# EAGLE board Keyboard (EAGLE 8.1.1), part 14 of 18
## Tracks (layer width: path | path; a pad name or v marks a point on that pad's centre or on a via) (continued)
S$14353
  Bottom 0: 155.42,84.92 155.38,84.86
S$14354
  Bottom 0: 155.38,84.86 155.35,84.8
S$14355
  Bottom 0: 155.35,84.8 155.34,84.73
S$14356
  Bottom 0: 155.34,84.73 155.33,84.66
S$14357
  Bottom 0: 155.33,84.66 155.33,76.26
S$14358
  Bottom 0: 155.33,76.26 155.24,76.17
S$14359
  Bottom 0: 155.24,76.17 155.06,75.89
S$14360
  Bottom 0: 155.06,75.89 154.98,75.58
S$14361
  Bottom 0: 154.98,75.58 154.98,75.26
S$14362
  Bottom 0: 154.98,75.26 155.06,74.94
S$14363
  Bottom 0: 155.06,74.94 155.24,74.67
S$14364
  Bottom 0: 155.24,74.67 155.47,74.44
S$14365
  Bottom 0: 155.47,74.44 155.76,74.3
S$14366
  Bottom 0: 155.76,74.3 156.08,74.23
S$14367
  Bottom 0: 156.08,74.23 156.41,74.25
S$14368
  Bottom 0: 156.41,74.25 156.71,74.36
S$14369
  Bottom 0: 156.71,74.36 156.97,74.55
S$14370
  Bottom 0: 156.97,74.55 157.18,74.8
S$14371
  Bottom 0: 157.18,74.8 157.31,75.1
S$14372
  Bottom 0: 157.31,75.1 157.36,75.42
S$14373
  Bottom 0: 157.36,75.42 157.31,75.74
S$14374
  Bottom 0: 157.31,75.74 157.18,76.04
S$14375
  Bottom 0: 157.18,76.04 156.97,76.29
S$14376
  Bottom 0: 156.97,76.29 156.71,76.48
S$14377
  Bottom 0: 156.71,76.48 156.41,76.59
S$14378
  Bottom 0: 156.41,76.59 156.22,76.6
S$14379
  Bottom 0: 156.22,76.6 156.22,77.98
S$14380
  Bottom 0: 156.22,77.98 156.29,77.85
S$14381
  Bottom 0: 156.29,77.85 156.53,77.6
S$14382
  Bottom 0: 156.53,77.6 156.82,77.41
S$14383
  Bottom 0: 156.82,77.41 157.15,77.31
S$14384
  Bottom 0: 157.15,77.31 157.5,77.28
S$14385
  Bottom 0: 157.5,77.28 157.85,77.35
S$14386
  Bottom 0: 157.85,77.35 158.16,77.5
S$14387
  Bottom 0: 158.16,77.5 158.43,77.72
S$14388
  Bottom 0: 158.43,77.72 158.64,78.01
S$14389
  Bottom 0: 158.64,78.01 158.77,78.33
S$14390
  Bottom 0: 158.77,78.33 158.81,78.68
S$14391
  Bottom 0: 158.81,78.68 158.77,79.02
S$14392
  Bottom 0: 158.77,79.02 158.64,79.35
S$14393
  Bottom 0: 158.64,79.35 158.43,79.63
S$14394
  Bottom 0: 158.43,79.63 158.16,79.86
S$14395
  Bottom 0: 158.16,79.86 157.85,80.01
S$14396
  Bottom 0: 157.85,80.01 157.5,80.07
S$14397
  Bottom 0: 157.5,80.07 157.15,80.05
S$14398
  Bottom 0: 157.15,80.05 156.82,79.94
S$14399
  Bottom 0: 156.82,79.94 156.53,79.75
S$14400
  Bottom 0: 156.53,79.75 156.29,79.5
S$14401
  Bottom 0: 156.29,79.5 156.22,79.37
S$14402
  Bottom 0: 156.22,79.37 156.22,84.48
S$14403
  Bottom 0: 156.22,84.48 159,87.25
S$14404
  Bottom 0: 159,87.25 159.03,87.31
S$14405
  Bottom 0: 159.03,87.31 159.07,87.35
S$14406
  Bottom 0: 159.07,87.35 159.08,87.39
S$14407
  Bottom 0: 159.08,87.39 159.11,87.45
S$14408
  Bottom 0: 159.11,87.45 159.11,87.51
S$14409
  Bottom 0: 159.11,87.51 159.13,87.57
S$14410
  Bottom 0: 159.13,87.57 159.13,87.69
S$14411
  Bottom 0: 159.13,87.69 159.58,87.69
S$14412
  Bottom 0: 159.58,87.69 159.65,87.7
S$14413
  Bottom 0: 159.65,87.7 159.72,87.74
S$14414
  Bottom 0: 159.72,87.74 159.78,87.8
S$14415
  Bottom 0: 159.78,87.8 159.82,87.87
S$14416
  Bottom 0: 159.82,87.87 159.83,87.95
S$14417
  Bottom 0: 159.83,87.95 159.83,89.65
S$14418
  Bottom 0: 159.83,89.65 160.44,89.65
S$14419
  Bottom 0: 160.44,89.65 160.27,89.46
S$14420
  Bottom 0: 160.27,89.46 160.13,89.16
S$14421
  Bottom 0: 160.13,89.16 160.08,88.84
S$14422
  Bottom 0: 160.08,88.84 160.13,88.52
S$14423
  Bottom 0: 160.13,88.52 160.27,88.22
S$14424
  Bottom 0: 160.27,88.22 160.48,87.97
S$14425
  Bottom 0: 160.48,87.97 160.75,87.8
S$14426
  Bottom 0: 160.75,87.8 161.06,87.7
S$14427
  Bottom 0: 161.06,87.7 161.39,87.7
S$14428
  Bottom 0: 161.39,87.7 161.52,87.74
S$14429
  Bottom 0: 161.52,87.74 161.91,87.35
S$14430
  Bottom 0: 161.91,87.35 161.91,84.92
S$14431
  Bottom 0: 161.91,84.92 161.86,85.03
S$14432
  Bottom 0: 161.86,85.03 161.57,85.37
S$14433
  Bottom 0: 161.57,85.37 161.23,85.66
S$14434
  Bottom 0: 161.23,85.66 160.83,85.87
S$14435
  Bottom 0: 160.83,85.87 160.4,86
S$14436
  Bottom 0: 160.4,86 159.96,86.04
S$14437
  Bottom 0: 159.96,86.04 159.51,86
S$14438
  Bottom 0: 159.51,86 159.08,85.87
S$14439
  Bottom 0: 159.08,85.87 158.69,85.66
S$14440
  Bottom 0: 158.69,85.66 158.34,85.37
S$14441
  Bottom 0: 158.34,85.37 158.06,85.03
S$14442
  Bottom 0: 158.06,85.03 157.84,84.63
S$14443
  Bottom 0: 157.84,84.63 157.71,84.2
S$14444
  Bottom 0: 157.71,84.2 157.67,83.76
S$14445
  Bottom 0: 157.67,83.76 157.71,83.31
S$14446
  Bottom 0: 157.71,83.31 157.84,82.88
S$14447
  Bottom 0: 157.84,82.88 158.06,82.49
S$14448
  Bottom 0: 158.06,82.49 158.34,82.14
S$14449
  Bottom 0: 158.34,82.14 158.69,81.86
S$14450
  Bottom 0: 158.69,81.86 159.08,81.64
S$14451
  Bottom 0: 159.08,81.64 159.51,81.52
S$14452
  Bottom 0: 159.51,81.52 159.96,81.47
S$14453
  Bottom 0: 159.96,81.47 160.4,81.52
S$14454
  Bottom 0: 160.4,81.52 160.83,81.64
S$14455
  Bottom 0: 160.83,81.64 161.23,81.86
S$14456
  Bottom 0: 161.23,81.86 161.43,82.02
S$14457
  Bottom 0: 161.43,82.02 161.43,73.36
S$14458
  Bottom 0: 161.43,73.36 161.43,73.27
S$14459
  Bottom 0: 161.43,73.27 161.45,73.19
S$14460
  Bottom 0: 161.45,73.19 161.49,73.1
S$14461
  Bottom 0: 161.49,73.1 161.53,73.03
S$14462
  Bottom 0: 161.53,73.03 161.59,72.96
S$14463
  Bottom 0: 161.59,72.96 166.56,68
S$14464
  Bottom 0: 166.56,68 166.62,67.94
S$14465
  Bottom 0: 166.62,67.94 166.7,67.89
S$14466
  Bottom 0: 166.7,67.89 166.78,67.86
S$14467
  Bottom 0: 166.78,67.86 166.87,67.83
S$14468
  Bottom 0: 166.87,67.83 166.96,67.83
S$14469
  Bottom 0: 166.96,67.83 169.37,67.83
S$14470
  Bottom 0: 169.37,67.83 169.46,67.83
S$14471
  Bottom 0: 169.46,67.83 169.54,67.86
S$14472
  Bottom 0: 169.54,67.86 169.62,67.89
S$14473
  Bottom 0: 169.62,67.89 169.7,67.94
S$14474
  Bottom 0: 169.7,67.94 169.76,68
S$14475
  Bottom 0: 169.76,68 170.46,68.69
S$14476
  Bottom 0: 170.46,68.69 170.59,68.65
S$14477
  Bottom 0: 170.59,68.65 170.91,68.65
S$14478
  Bottom 0: 170.91,68.65 171.22,68.75
S$14479
  Bottom 0: 171.22,68.75 171.5,68.92
S$14480
  Bottom 0: 171.5,68.92 171.71,69.16
S$14481
  Bottom 0: 171.71,69.16 171.85,69.47
S$14482
  Bottom 0: 171.85,69.47 171.89,69.79
S$14483
  Bottom 0: 171.89,69.79 171.85,70.11
S$14484
  Bottom 0: 171.85,70.11 171.71,70.41
S$14485
  Bottom 0: 171.71,70.41 171.5,70.65
S$14486
  Bottom 0: 171.5,70.65 171.22,70.83
S$14487
  Bottom 0: 171.22,70.83 170.91,70.92
S$14488
  Bottom 0: 170.91,70.92 170.59,70.92
S$14489
  Bottom 0: 170.59,70.92 170.28,70.83
S$14490
  Bottom 0: 170.28,70.83 170,70.65
S$14491
  Bottom 0: 170,70.65 169.79,70.41
S$14492
  Bottom 0: 169.79,70.41 169.65,70.11
S$14493
  Bottom 0: 169.65,70.11 169.61,69.79
S$14494
  Bottom 0: 169.61,69.79 169.65,69.48
S$14495
  Bottom 0: 169.65,69.48 169.35,69.19
S$14496
  Bottom 0: 169.35,69.19 169.35,70.67
S$14497
  Bottom 0: 169.35,70.67 169.34,70.75
S$14498
  Bottom 0: 169.34,70.75 169.3,70.82
S$14499
  Bottom 0: 169.3,70.82 169.25,70.88
S$14500
  Bottom 0: 169.25,70.88 169.18,70.92
S$14501
  Bottom 0: 169.18,70.92 169.1,70.93
S$14502
  Bottom 0: 169.1,70.93 168.65,70.93
S$14503
  Bottom 0: 168.65,70.93 168.65,71.06
S$14504
  Bottom 0: 168.65,71.06 168.59,71.28
S$14505
  Bottom 0: 168.59,71.28 168.43,71.44
S$14506
  Bottom 0: 168.43,71.44 168.21,71.5
S$14507
  Bottom 0: 168.21,71.5 167.86,71.5
S$14508
  Bottom 0: 167.86,71.5 166.77,72.58
S$14509
  Bottom 0: 166.77,72.58 166.84,72.72
S$14510
  Bottom 0: 166.84,72.72 166.88,73.04
S$14511
  Bottom 0: 166.88,73.04 166.84,73.36
S$14512
  Bottom 0: 166.84,73.36 166.71,73.66
S$14513
  Bottom 0: 166.71,73.66 166.5,73.92
S$14514
  Bottom 0: 166.5,73.92 166.24,74.11
S$14515
  Bottom 0: 166.24,74.11 165.93,74.21
S$14516
  Bottom 0: 165.93,74.21 165.6,74.23
S$14517
  Bottom 0: 165.6,74.23 165.28,74.17
S$14518
  Bottom 0: 165.28,74.17 165,74.02
S$14519
  Bottom 0: 165,74.02 164.76,73.8
S$14520
  Bottom 0: 164.76,73.8 164.59,73.52
S$14521
  Bottom 0: 164.59,73.52 164.5,73.2
S$14522
  Bottom 0: 164.5,73.2 164.5,72.88
S$14523
  Bottom 0: 164.5,72.88 164.59,72.56
S$14524
  Bottom 0: 164.59,72.56 164.76,72.29
S$14525
  Bottom 0: 164.76,72.29 165,72.07
S$14526
  Bottom 0: 165,72.07 165.28,71.92
S$14527
  Bottom 0: 165.28,71.92 165.6,71.85
S$14528
  Bottom 0: 165.6,71.85 165.93,71.87
S$14529
  Bottom 0: 165.93,71.87 166.15,71.95
S$14530
  Bottom 0: 166.15,71.95 167.21,70.9
S$14531
  Bottom 0: 167.21,70.9 167.18,70.88
S$14532
  Bottom 0: 167.18,70.88 167.12,70.82
S$14533
  Bottom 0: 167.12,70.82 167.08,70.75
S$14534
  Bottom 0: 167.08,70.75 167.07,70.67
S$14535
  Bottom 0: 167.07,70.67 167.07,69.09
S$14536
  Bottom 0: 167.07,69.09 162.56,73.6
S$14537
  Bottom 0: 162.56,73.6 162.56,80.53
S$14538
  Bottom 0: 162.56,80.53 162.64,80.39
S$14539
  Bottom 0: 162.64,80.39 162.88,80.14
S$14540
  Bottom 0: 162.88,80.14 163.17,79.95
S$14541
  Bottom 0: 163.17,79.95 163.5,79.84
S$14542
  Bottom 0: 163.5,79.84 163.85,79.83
S$14543
  Bottom 0: 163.85,79.83 164.2,79.89
S$14544
  Bottom 0: 164.2,79.89 164.38,79.97
S$14545
  Bottom 0: 164.38,79.97 167.75,76.6
S$14546
  Bottom 0: 167.75,76.6 167.81,76.56
S$14547
  Bottom 0: 167.81,76.56 167.87,76.52
S$14548
  Bottom 0: 167.87,76.52 167.93,76.5
S$14549
  Bottom 0: 167.93,76.5 167.99,76.48
S$14550
  Bottom 0: 167.99,76.48 168.06,76.48
S$14551
  Bottom 0: 168.06,76.48 171.65,76.48
S$14552
  Bottom 0: 171.65,76.48 174.33,73.79
S$14553
  Bottom 0: 174.33,73.79 174.39,73.75
S$14554
  Bottom 0: 174.39,73.75 174.45,73.71
S$14555
  Bottom 0: 174.45,73.71 174.51,73.68
S$14556
  Bottom 0: 174.51,73.68 174.58,73.67
S$14557
  Bottom 0: 174.58,73.67 174.65,73.66
S$14558
  Bottom 0: 174.65,73.66 178.43,73.66
S$14559
  Bottom 0: 178.43,73.66 178.5,73.67
S$14560
  Bottom 0: 178.5,73.67 178.57,73.68
S$14561
  Bottom 0: 178.57,73.68 178.63,73.71
S$14562
  Bottom 0: 178.63,73.71 178.69,73.75
S$14563
  Bottom 0: 178.69,73.75 178.75,73.79
S$14564
  Bottom 0: 178.75,73.79 181.28,76.32
S$14565
  Bottom 0: 181.28,76.32 182.07,76.32
S$14566
  Bottom 0: 182.07,76.32 181.91,76.17
S$14567
  Bottom 0: 181.91,76.17 181.74,75.89
S$14568
  Bottom 0: 181.74,75.89 181.65,75.58
S$14569
  Bottom 0: 181.65,75.58 181.65,75.25
S$14570
  Bottom 0: 181.65,75.25 181.7,75.08
S$14571
  Bottom 0: 181.7,75.08 180.23,73.61
S$14572
  Bottom 0: 180.23,73.61 174.35,73.61
S$14573
  Bottom 0: 174.35,73.61 174.33,73.66
S$14574
  Bottom 0: 174.33,73.66 174.12,73.92
S$14575
  Bottom 0: 174.12,73.92 173.85,74.11
S$14576
  Bottom 0: 173.85,74.11 173.55,74.21
S$14577
  Bottom 0: 173.55,74.21 173.22,74.23
S$14578
  Bottom 0: 173.22,74.23 172.98,74.18
S$14579
  Bottom 0: 172.98,74.18 171.34,75.82
S$14580
  Bottom 0: 171.34,75.82 171.27,75.88
S$14581
  Bottom 0: 171.27,75.88 171.19,75.93
S$14582
  Bottom 0: 171.19,75.93 171.11,75.96
S$14583
  Bottom 0: 171.11,75.96 171.03,75.98
S$14584
  Bottom 0: 171.03,75.98 170.93,75.99
S$14585
  Bottom 0: 170.93,75.99 164.82,75.99
S$14586
  Bottom 0: 164.82,75.99 164.8,76.04
S$14587
  Bottom 0: 164.8,76.04 164.59,76.29
S$14588
  Bottom 0: 164.59,76.29 164.33,76.48
S$14589
  Bottom 0: 164.33,76.48 164.03,76.59
S$14590
  Bottom 0: 164.03,76.59 163.7,76.61
S$14591
  Bottom 0: 163.7,76.61 163.38,76.54
S$14592
  Bottom 0: 163.38,76.54 163.09,76.4
S$14593
  Bottom 0: 163.09,76.4 162.85,76.17
S$14594
  Bottom 0: 162.85,76.17 162.68,75.89
S$14595
  Bottom 0: 162.68,75.89 162.6,75.58
S$14596
  Bottom 0: 162.6,75.58 162.6,75.26
S$14597
  Bottom 0: 162.6,75.26 162.68,74.94
S$14598
  Bottom 0: 162.68,74.94 162.85,74.67
S$14599
  Bottom 0: 162.85,74.67 163.09,74.44
S$14600
  Bottom 0: 163.09,74.44 163.38,74.3
S$14601
  Bottom 0: 163.38,74.3 163.7,74.23
S$14602
  Bottom 0: 163.7,74.23 164.03,74.25
S$14603
  Bottom 0: 164.03,74.25 164.33,74.36
S$14604
  Bottom 0: 164.33,74.36 164.59,74.55
S$14605
  Bottom 0: 164.59,74.55 164.8,74.8
S$14606
  Bottom 0: 164.8,74.8 164.82,74.85
S$14607
  Bottom 0: 164.82,74.85 170.7,74.85
S$14608
  Bottom 0: 170.7,74.85 172.17,73.38
S$14609
  Bottom 0: 172.17,73.38 172.12,73.2
S$14610
  Bottom 0: 172.12,73.2 172.12,72.88
S$14611
  Bottom 0: 172.12,72.88 172.21,72.56
S$14612
  Bottom 0: 172.21,72.56 172.38,72.29
S$14613
  Bottom 0: 172.38,72.29 172.61,72.07
S$14614
  Bottom 0: 172.61,72.07 172.91,71.92
S$14615
  Bottom 0: 172.91,71.92 173.22,71.85
S$14616
  Bottom 0: 173.22,71.85 173.55,71.87
S$14617
  Bottom 0: 173.55,71.87 173.85,71.98
S$14618
  Bottom 0: 173.85,71.98 174.12,72.17
S$14619
  Bottom 0: 174.12,72.17 174.33,72.42
S$14620
  Bottom 0: 174.33,72.42 174.35,72.47
S$14621
  Bottom 0: 174.35,72.47 180.46,72.47
S$14622
  Bottom 0: 180.46,72.47 180.55,72.48
S$14623
  Bottom 0: 180.55,72.48 180.64,72.5
S$14624
  Bottom 0: 180.64,72.5 180.72,72.53
S$14625
  Bottom 0: 180.72,72.53 180.8,72.58
S$14626
  Bottom 0: 180.8,72.58 180.87,72.64
S$14627
  Bottom 0: 180.87,72.64 182.5,74.28
S$14628
  Bottom 0: 182.5,74.28 182.76,74.23
S$14629
  Bottom 0: 182.76,74.23 183.08,74.24
S$14630
  Bottom 0: 183.08,74.24 183.38,74.35
S$14631
  Bottom 0: 183.38,74.35 183.65,74.54
S$14632
  Bottom 0: 183.65,74.54 183.85,74.8
S$14633
  Bottom 0: 183.85,74.8 183.88,74.84
S$14634
  Bottom 0: 183.88,74.84 189.76,74.84
S$14635
  Bottom 0: 189.76,74.84 191.22,73.38
S$14636
  Bottom 0: 191.22,73.38 191.18,73.2
S$14637
  Bottom 0: 191.18,73.2 191.18,72.88
S$14638
  Bottom 0: 191.18,72.88 191.26,72.56
S$14639
  Bottom 0: 191.26,72.56 191.44,72.29
S$14640
  Bottom 0: 191.44,72.29 191.67,72.07
S$14641
  Bottom 0: 191.67,72.07 191.96,71.92
S$14642
  Bottom 0: 191.96,71.92 192.28,71.85
S$14643
  Bottom 0: 192.28,71.85 192.61,71.87
S$14644
  Bottom 0: 192.61,71.87 192.91,71.98
S$14645
  Bottom 0: 192.91,71.98 193.18,72.17
S$14646
  Bottom 0: 193.18,72.17 193.38,72.42
S$14647
  Bottom 0: 193.38,72.42 193.51,72.72
S$14648
  Bottom 0: 193.51,72.72 193.56,73.04
S$14649
  Bottom 0: 193.56,73.04 193.52,73.29
S$14650
  Bottom 0: 193.52,73.29 194.4,72.41
S$14651
  Bottom 0: 194.4,72.41 194.46,72.37
S$14652
  Bottom 0: 194.46,72.37 194.52,72.33
S$14653
  Bottom 0: 194.52,72.33 194.58,72.3
S$14654
  Bottom 0: 194.58,72.3 194.64,72.29
S$14655
  Bottom 0: 194.64,72.29 194.71,72.28
S$14656
  Bottom 0: 194.71,72.28 200.03,72.28
S$14657
  Bottom 0: 200.03,72.28 204.76,67.55
S$14658
  Bottom 0: 204.76,67.55 204.81,67.51
S$14659
  Bottom 0: 204.81,67.51 204.87,67.47
S$14660
  Bottom 0: 204.87,67.47 204.94,67.44
S$14661
  Bottom 0: 204.94,67.44 205,67.43
S$14662
  Bottom 0: 205,67.43 205.07,67.42
S$14663
  Bottom 0: 205.07,67.42 207.63,67.42
S$14664
  Bottom 0: 207.63,67.42 208.13,66.92
S$14665
  Bottom 0: 208.13,66.92 208.03,66.94
S$14666
  Bottom 0: 208.03,66.94 207.58,66.99
S$14667
  Bottom 0: 207.58,66.99 207.13,66.94
S$14668
  Bottom 0: 207.13,66.94 206.71,66.82
S$14669
  Bottom 0: 206.71,66.82 206.31,66.61
S$14670
  Bottom 0: 206.31,66.61 205.97,66.32
S$14671
  Bottom 0: 205.97,66.32 205.68,65.98
S$14672
  Bottom 0: 205.68,65.98 205.47,65.58
S$14673
  Bottom 0: 205.47,65.58 205.34,65.15
S$14674
  Bottom 0: 205.34,65.15 205.3,64.71
S$14675
  Bottom 0: 205.3,64.71 205.34,64.26
S$14676
  Bottom 0: 205.34,64.26 205.47,63.83
S$14677
  Bottom 0: 205.47,63.83 205.68,63.44
S$14678
  Bottom 0: 205.68,63.44 205.97,63.09
S$14679
  Bottom 0: 205.97,63.09 206.31,62.81
S$14680
  Bottom 0: 206.31,62.81 206.71,62.59
S$14681
  Bottom 0: 206.71,62.59 207.13,62.47
S$14682
  Bottom 0: 207.13,62.47 207.58,62.42
S$14683
  Bottom 0: 207.58,62.42 208.03,62.47
S$14684
  Bottom 0: 208.03,62.47 208.46,62.59
S$14685
  Bottom 0: 208.46,62.59 208.85,62.81
S$14686
  Bottom 0: 208.85,62.81 209.19,63.09
S$14687
  Bottom 0: 209.19,63.09 209.48,63.44
S$14688
  Bottom 0: 209.48,63.44 209.69,63.83
S$14689
  Bottom 0: 209.69,63.83 209.82,64.26
S$14690
  Bottom 0: 209.82,64.26 209.87,64.71
S$14691
  Bottom 0: 209.87,64.71 209.82,65.15
S$14692
  Bottom 0: 209.82,65.15 209.79,65.26
S$14693
  Bottom 0: 209.79,65.26 211.5,63.55
S$14694
  Bottom 0: 211.5,63.55 211.47,63.56
S$14695
  Bottom 0: 211.47,63.56 211.13,63.54
S$14696
  Bottom 0: 211.13,63.54 210.8,63.43
S$14697
  Bottom 0: 210.8,63.43 210.5,63.24
S$14698
  Bottom 0: 210.5,63.24 210.26,62.99
S$14699
  Bottom 0: 210.26,62.99 210.09,62.68
S$14700
  Bottom 0: 210.09,62.68 210,62.34
S$14701
  Bottom 0: 210,62.34 210,61.99
S$14702
  Bottom 0: 210,61.99 210.09,61.65
S$14703
  Bottom 0: 210.09,61.65 210.26,61.34
S$14704
  Bottom 0: 210.26,61.34 210.5,61.09
S$14705
  Bottom 0: 210.5,61.09 210.8,60.9
S$14706
  Bottom 0: 210.8,60.9 211.13,60.8
S$14707
  Bottom 0: 211.13,60.8 211.47,60.77
S$14708
  Bottom 0: 211.47,60.77 211.82,60.84
S$14709
  Bottom 0: 211.82,60.84 212.14,60.99
S$14710
  Bottom 0: 212.14,60.99 212.41,61.21
S$14711
  Bottom 0: 212.41,61.21 212.62,61.5
S$14712
  Bottom 0: 212.62,61.5 212.74,61.82
S$14713
  Bottom 0: 212.74,61.82 212.79,62.17
S$14714
  Bottom 0: 212.79,62.17 212.77,62.28
S$14715
  Bottom 0: 212.77,62.28 223.37,51.68
S$14716
  Bottom 0: 223.37,51.68 223.43,51.64
S$14717
  Bottom 0: 223.43,51.64 223.48,51.6
S$14718
  Bottom 0: 223.48,51.6 223.54,51.57
S$14719
  Bottom 0: 223.54,51.57 223.61,51.56
S$14720
  Bottom 0: 223.61,51.56 223.69,51.55
S$14721
  Bottom 0: 223.69,51.55 228.98,51.55
S$14722
  Bottom 0: 228.98,51.55 228.98,49.84
S$14723
  Bottom 0: 228.98,49.84 222.88,49.84
S$14724
  Bottom 0: 222.88,49.84 222.86,50
S$14725
  Bottom 0: 222.86,50 222.72,50.27
S$14726
  Bottom 0: 222.72,50.27 222.52,50.49
S$14727
  Bottom 0: 222.52,50.49 222.26,50.65
S$14728
  Bottom 0: 222.26,50.65 221.96,50.71
S$14729
  Bottom 0: 221.96,50.71 221.66,50.69
S$14730
  Bottom 0: 221.66,50.69 221.38,50.58
S$14731
  Bottom 0: 221.38,50.58 221.14,50.39
S$14732
  Bottom 0: 221.14,50.39 220.97,50.14
S$14733
  Bottom 0: 220.97,50.14 220.88,49.85
S$14734
  Bottom 0: 220.88,49.85 220.88,49.55
S$14735
  Bottom 0: 220.88,49.55 220.97,49.26
S$14736
  Bottom 0: 220.97,49.26 221.14,49.01
S$14737
  Bottom 0: 221.14,49.01 221.38,48.82
S$14738
  Bottom 0: 221.38,48.82 221.66,48.71
S$14739
  Bottom 0: 221.66,48.71 221.96,48.69
S$14740
  Bottom 0: 221.96,48.69 222.26,48.76
S$14741
  Bottom 0: 222.26,48.76 222.52,48.91
S$14742
  Bottom 0: 222.52,48.91 222.56,48.95
S$14743
  Bottom 0: 222.56,48.95 240.27,48.95
S$14744
  Bottom 0: 240.27,48.95 240.43,48.82
S$14745
  Bottom 0: 240.43,48.82 240.71,48.71
S$14746
  Bottom 0: 240.71,48.71 241.02,48.69
S$14747
  Bottom 0: 241.02,48.69 241.31,48.76
S$14748
  Bottom 0: 241.31,48.76 241.57,48.91
S$14749
  Bottom 0: 241.57,48.91 241.78,49.13
S$14750
  Bottom 0: 241.78,49.13 241.91,49.4
S$14751
  Bottom 0: 241.91,49.4 241.96,49.7
S$14752
  Bottom 0: 241.96,49.7 241.91,50
S$14753
  Bottom 0: 241.91,50 241.78,50.27
S$14754
  Bottom 0: 241.78,50.27 241.57,50.49
S$14755
  Bottom 0: 241.57,50.49 241.31,50.65
S$14756
  Bottom 0: 241.31,50.65 241.02,50.71
S$14757
  Bottom 0: 241.02,50.71 240.71,50.69
S$14758
  Bottom 0: 240.71,50.69 240.43,50.58
S$14759
  Bottom 0: 240.43,50.58 240.19,50.39
S$14760
  Bottom 0: 240.19,50.39 240.03,50.14
S$14761
  Bottom 0: 240.03,50.14 239.94,49.85
S$14762
  Bottom 0: 239.94,49.85 239.94,49.84
S$14763
  Bottom 0: 239.94,49.84 233.35,49.84
S$14764
  Bottom 0: 233.35,49.84 233.41,49.87
S$14765
  Bottom 0: 233.41,49.87 233.62,50.11
S$14766
  Bottom 0: 233.62,50.11 233.76,50.42
S$14767
  Bottom 0: 233.76,50.42 233.8,50.74
S$14768
  Bottom 0: 233.8,50.74 233.76,51.06
S$14769
  Bottom 0: 233.76,51.06 233.62,51.36
S$14770
  Bottom 0: 233.62,51.36 233.45,51.55
S$14771
  Bottom 0: 233.45,51.55 240.78,51.55
S$14772
  Bottom 0: 240.78,51.55 242.49,49.84
S$14773
  Bottom 0: 242.49,49.84 242.49,49.67
S$14774
  Bottom 0: 242.49,49.67 242.53,49.54
S$14775
  Bottom 0: 242.53,49.54 242.43,49.53
S$14776
  Bottom 0: 242.43,49.53 242.21,49.41
S$14777
  Bottom 0: 242.21,49.41 242.03,49.23
S$14778
  Bottom 0: 242.03,49.23 241.94,48.99
S$14779
  Bottom 0: 241.94,48.99 241.94,48.74
S$14780
  Bottom 0: 241.94,48.74 242.03,48.51
S$14781
  Bottom 0: 242.03,48.51 242.08,48.46
S$14782
  Bottom 0: 242.08,48.46 236.58,42.96
S$14783
  Bottom 0: 179.09,67.74 179.39,67.81
S$14784
  Bottom 0: 179.39,67.81 179.66,67.95
S$14785
  Bottom 0: 179.66,67.95 179.86,68.18
S$14786
  Bottom 0: 179.86,68.18 179.99,68.45
S$14787
  Bottom 0: 179.99,68.45 180.04,68.75
S$14788
  Bottom 0: 180.04,68.75 179.99,69.05
S$14789
  Bottom 0: 179.99,69.05 179.86,69.32
S$14790
  Bottom 0: 179.86,69.32 179.66,69.54
S$14791
  Bottom 0: 179.66,69.54 179.39,69.69
S$14792
  Bottom 0: 179.39,69.69 179.09,69.76
S$14793
  Bottom 0: 179.09,69.76 178.79,69.74
S$14794
  Bottom 0: 178.79,69.74 178.51,69.63
S$14795
  Bottom 0: 178.51,69.63 178.27,69.44
S$14796
  Bottom 0: 178.27,69.44 178.11,69.19
S$14797
  Bottom 0: 178.11,69.19 178.01,68.9
S$14798
  Bottom 0: 178.01,68.9 178.01,68.59
S$14799
  Bottom 0: 178.01,68.59 178.11,68.31
S$14800
  Bottom 0: 178.11,68.31 178.27,68.06
S$14801
  Bottom 0: 178.27,68.06 178.51,67.87
S$14802
  Bottom 0: 178.51,67.87 178.79,67.76
S$14803
  Bottom 0: 178.79,67.76 179.09,67.74
S$14804
  Bottom 0: 160.05,67.74 160.34,67.81
S$14805
  Bottom 0: 160.34,67.81 160.6,67.95
S$14806
  Bottom 0: 160.6,67.95 160.81,68.18
S$14807
  Bottom 0: 160.81,68.18 160.94,68.45
S$14808
  Bottom 0: 160.94,68.45 160.99,68.75
S$14809
  Bottom 0: 160.99,68.75 160.94,69.05
S$14810
  Bottom 0: 160.94,69.05 160.81,69.32
S$14811
  Bottom 0: 160.81,69.32 160.6,69.54
S$14812
  Bottom 0: 160.6,69.54 160.34,69.69
S$14813
  Bottom 0: 160.34,69.69 160.05,69.76
S$14814
  Bottom 0: 160.05,69.76 159.74,69.74
S$14815
  Bottom 0: 159.74,69.74 159.46,69.63
S$14816
  Bottom 0: 159.46,69.63 159.22,69.44
S$14817
  Bottom 0: 159.22,69.44 159.06,69.19
S$14818
  Bottom 0: 159.06,69.19 158.97,68.9
S$14819
  Bottom 0: 158.97,68.9 158.97,68.59
S$14820
  Bottom 0: 158.97,68.59 159.06,68.31
S$14821
  Bottom 0: 159.06,68.31 159.22,68.06
S$14822
  Bottom 0: 159.22,68.06 159.46,67.87
S$14823
  Bottom 0: 159.46,67.87 159.74,67.76
S$14824
  Bottom 0: 159.74,67.76 160.05,67.74
S$14825
  Bottom 0: 186.37,68.64 188.15,68.64
S$14826
  Bottom 0: 188.15,68.64 188.23,68.65
S$14827
  Bottom 0: 188.23,68.65 188.3,68.69
S$14828
  Bottom 0: 188.3,68.69 188.35,68.75
S$14829
  Bottom 0: 188.35,68.75 188.39,68.82
S$14830
  Bottom 0: 188.39,68.82 188.41,68.9
S$14831
  Bottom 0: 188.41,68.9 188.41,70.67
S$14832
  Bottom 0: 188.41,70.67 188.39,70.75
S$14833
  Bottom 0: 188.39,70.75 188.35,70.82
S$14834
  Bottom 0: 188.35,70.82 188.3,70.88
S$14835
  Bottom 0: 188.3,70.88 188.23,70.92
S$14836
  Bottom 0: 188.23,70.92 188.15,70.93
S$14837
  Bottom 0: 188.15,70.93 187.7,70.93
S$14838
  Bottom 0: 187.7,70.93 187.7,71.06
S$14839
  Bottom 0: 187.7,71.06 187.64,71.28
S$14840
  Bottom 0: 187.64,71.28 187.48,71.44
S$14841
  Bottom 0: 187.48,71.44 187.26,71.5
S$14842
  Bottom 0: 187.26,71.5 186.92,71.5
S$14843
  Bottom 0: 186.92,71.5 185.83,72.59
S$14844
  Bottom 0: 185.83,72.59 185.89,72.72
S$14845
  Bottom 0: 185.89,72.72 185.94,73.04
S$14846
  Bottom 0: 185.94,73.04 185.89,73.36
S$14847
  Bottom 0: 185.89,73.36 185.76,73.66
S$14848
  Bottom 0: 185.76,73.66 185.56,73.92
S$14849
  Bottom 0: 185.56,73.92 185.29,74.11
S$14850
  Bottom 0: 185.29,74.11 184.99,74.21
S$14851
  Bottom 0: 184.99,74.21 184.66,74.23
S$14852
  Bottom 0: 184.66,74.23 184.34,74.17
S$14853
  Bottom 0: 184.34,74.17 184.05,74.02
S$14854
  Bottom 0: 184.05,74.02 183.82,73.8
S$14855
  Bottom 0: 183.82,73.8 183.65,73.52
S$14856
  Bottom 0: 183.65,73.52 183.56,73.2
S$14857
  Bottom 0: 183.56,73.2 183.56,72.88
S$14858
  Bottom 0: 183.56,72.88 183.65,72.56
S$14859
  Bottom 0: 183.65,72.56 183.82,72.29
S$14860
  Bottom 0: 183.82,72.29 184.05,72.07
S$14861
  Bottom 0: 184.05,72.07 184.34,71.92
S$14862
  Bottom 0: 184.34,71.92 184.66,71.85
S$14863
  Bottom 0: 184.66,71.85 184.99,71.87
S$14864
  Bottom 0: 184.99,71.87 185.2,71.95
S$14865
  Bottom 0: 185.2,71.95 186.26,70.9
S$14866
  Bottom 0: 186.26,70.9 186.22,70.88
S$14867
  Bottom 0: 186.22,70.88 186.17,70.82
S$14868
  Bottom 0: 186.17,70.82 186.13,70.75
S$14869
  Bottom 0: 186.13,70.75 186.12,70.67
S$14870
  Bottom 0: 186.12,70.67 186.12,68.9
S$14871
  Bottom 0: 186.12,68.9 186.13,68.82
S$14872
  Bottom 0: 186.13,68.82 186.17,68.75
S$14873
  Bottom 0: 186.17,68.75 186.22,68.69
S$14874
  Bottom 0: 186.22,68.69 186.3,68.65
S$14875
  Bottom 0: 186.3,68.65 186.37,68.64
S$14876
  Bottom 0: 189.64,68.65 189.96,68.65
S$14877
  Bottom 0: 189.96,68.65 190.27,68.75
S$14878
  Bottom 0: 190.27,68.75 190.55,68.92
S$14879
  Bottom 0: 190.55,68.92 190.76,69.16
S$14880
  Bottom 0: 190.76,69.16 190.9,69.47
S$14881
  Bottom 0: 190.9,69.47 190.94,69.79
S$14882
  Bottom 0: 190.94,69.79 190.9,70.11
S$14883
  Bottom 0: 190.9,70.11 190.76,70.41
S$14884
  Bottom 0: 190.76,70.41 190.55,70.65
S$14885
  Bottom 0: 190.55,70.65 190.27,70.83
S$14886
  Bottom 0: 190.27,70.83 189.96,70.92
S$14887
  Bottom 0: 189.96,70.92 189.64,70.92
S$14888
  Bottom 0: 189.64,70.92 189.33,70.83
S$14889
  Bottom 0: 189.33,70.83 189.06,70.65
S$14890
  Bottom 0: 189.06,70.65 188.84,70.41
S$14891
  Bottom 0: 188.84,70.41 188.7,70.11
S$14892
  Bottom 0: 188.7,70.11 188.66,69.79
S$14893
  Bottom 0: 188.66,69.79 188.7,69.47
S$14894
  Bottom 0: 188.7,69.47 188.84,69.16
S$14895
  Bottom 0: 188.84,69.16 189.06,68.92
S$14896
  Bottom 0: 189.06,68.92 189.33,68.75
S$14897
  Bottom 0: 189.33,68.75 189.64,68.65
S$14898
  Bottom 0: 150.52,79.17 150.82,79.24
S$14899
  Bottom 0: 150.82,79.24 151.08,79.39
S$14900
  Bottom 0: 151.08,79.39 151.28,79.61
S$14901
  Bottom 0: 151.28,79.61 151.42,79.89
S$14902
  Bottom 0: 151.42,79.89 151.46,80.19
S$14903
  Bottom 0: 151.46,80.19 151.42,80.48
S$14904
  Bottom 0: 151.42,80.48 151.28,80.76
S$14905
  Bottom 0: 151.28,80.76 151.08,80.98
S$14906
  Bottom 0: 151.08,80.98 150.82,81.13
S$14907
  Bottom 0: 150.82,81.13 150.52,81.2
S$14908
  Bottom 0: 150.52,81.2 150.22,81.18
S$14909
  Bottom 0: 150.22,81.18 149.94,81.06
S$14910
  Bottom 0: 149.94,81.06 149.7,80.88
S$14911
  Bottom 0: 149.7,80.88 149.53,80.63
S$14912
  Bottom 0: 149.53,80.63 149.44,80.34
S$14913
  Bottom 0: 149.44,80.34 149.44,80.03
S$14914
  Bottom 0: 149.44,80.03 149.53,79.74
S$14915
  Bottom 0: 149.53,79.74 149.7,79.49
S$14916
  Bottom 0: 149.7,79.49 149.94,79.31
S$14917
  Bottom 0: 149.94,79.31 150.22,79.19
S$14918
  Bottom 0: 150.22,79.19 150.52,79.17
S$14919
  Bottom 0: 140.91,81.47 141.35,81.52
S$14920
  Bottom 0: 141.35,81.52 141.78,81.64
S$14921
  Bottom 0: 141.78,81.64 142.18,81.86
S$14922
  Bottom 0: 142.18,81.86 142.52,82.14
S$14923
  Bottom 0: 142.52,82.14 142.81,82.49
S$14924
  Bottom 0: 142.81,82.49 143.02,82.88
S$14925
  Bottom 0: 143.02,82.88 143.15,83.31
S$14926
  Bottom 0: 143.15,83.31 143.19,83.76
S$14927
  Bottom 0: 143.19,83.76 143.15,84.2
S$14928
  Bottom 0: 143.15,84.2 143.02,84.63
S$14929
  Bottom 0: 143.02,84.63 142.81,85.03
S$14930
  Bottom 0: 142.81,85.03 142.52,85.37
S$14931
  Bottom 0: 142.52,85.37 142.18,85.66
S$14932
  Bottom 0: 142.18,85.66 141.78,85.87
S$14933
  Bottom 0: 141.78,85.87 141.35,86
S$14934
  Bottom 0: 141.35,86 140.91,86.04
S$14935
  Bottom 0: 140.91,86.04 140.46,86
S$14936
  Bottom 0: 140.46,86 140.03,85.87
S$14937
  Bottom 0: 140.03,85.87 139.64,85.66
S$14938
  Bottom 0: 139.64,85.66 139.29,85.37
S$14939
  Bottom 0: 139.29,85.37 139.01,85.03
S$14940
  Bottom 0: 139.01,85.03 138.79,84.63
S$14941
  Bottom 0: 138.79,84.63 138.66,84.2
S$14942
  Bottom 0: 138.66,84.2 138.62,83.76
S$14943
  Bottom 0: 138.62,83.76 138.66,83.31
S$14944
  Bottom 0: 138.66,83.31 138.79,82.88
S$14945
  Bottom 0: 138.79,82.88 139.01,82.49
S$14946
  Bottom 0: 139.01,82.49 139.29,82.14
S$14947
  Bottom 0: 139.29,82.14 139.64,81.86
S$14948
  Bottom 0: 139.64,81.86 140.03,81.64
S$14949
  Bottom 0: 140.03,81.64 140.46,81.52
S$14950
  Bottom 0: 140.46,81.52 140.91,81.47
S$14951
  Bottom 0: 150.52,86.79 150.82,86.86
S$14952
  Bottom 0: 150.82,86.86 151.08,87.01
S$14953
  Bottom 0: 151.08,87.01 151.28,87.23
S$14954
  Bottom 0: 151.28,87.23 151.42,87.51
S$14955
  Bottom 0: 151.42,87.51 151.46,87.81
S$14956
  Bottom 0: 151.46,87.81 151.42,88.11
S$14957
  Bottom 0: 151.42,88.11 151.28,88.38
S$14958
  Bottom 0: 151.28,88.38 151.08,88.6
S$14959
  Bottom 0: 151.08,88.6 150.82,88.75
S$14960
  Bottom 0: 150.82,88.75 150.52,88.82
S$14961
  Bottom 0: 150.52,88.82 150.22,88.8
S$14962
  Bottom 0: 150.22,88.8 149.94,88.68
S$14963
  Bottom 0: 149.94,88.68 149.7,88.5
S$14964
  Bottom 0: 149.7,88.5 149.53,88.25
S$14965
  Bottom 0: 149.53,88.25 149.44,87.96
S$14966
  Bottom 0: 149.44,87.96 149.44,87.65
S$14967
  Bottom 0: 149.44,87.65 149.53,87.36
S$14968
  Bottom 0: 149.53,87.36 149.7,87.11
S$14969
  Bottom 0: 149.7,87.11 149.94,86.93
S$14970
  Bottom 0: 149.94,86.93 150.22,86.81
S$14971
  Bottom 0: 150.22,86.81 150.52,86.79
S$14972
  Bottom 0: 76.84,44.92 67.36,54.39
S$14973
  Bottom 0: 67.36,54.39 67.3,54.45
S$14974
  Bottom 0: 67.3,54.45 67.22,54.49
S$14975
  Bottom 0: 67.22,54.49 67.14,54.53
S$14976
  Bottom 0: 67.14,54.53 67.05,54.55
S$14977
  Bottom 0: 67.05,54.55 66.96,54.56
S$14978
  Bottom 0: 66.96,54.56 64.8,54.56
S$14979
  Bottom 0: 64.8,54.56 64.78,54.61
S$14980
  Bottom 0: 64.78,54.61 64.57,54.86
S$14981
  Bottom 0: 64.57,54.86 64.31,55.05
S$14982
  Bottom 0: 64.31,55.05 64,55.16
S$14983
  Bottom 0: 64,55.16 63.68,55.18
S$14984
  Bottom 0: 63.68,55.18 63.43,55.13
S$14985
  Bottom 0: 63.43,55.13 62.71,55.83
S$14986
  Bottom 0: 62.71,55.83 72.39,55.83
S$14987
  Bottom 0: 72.39,55.83 72.47,55.84
S$14988
  Bottom 0: 72.47,55.84 72.53,55.86
S$14989
  Bottom 0: 72.53,55.86 72.59,55.88
S$14990
  Bottom 0: 72.59,55.88 72.65,55.92
S$14991
  Bottom 0: 72.65,55.92 72.71,55.96
S$14992
  Bottom 0: 72.71,55.96 74.51,57.77
S$14993
  Bottom 0: 74.51,57.77 80.41,51.87
S$14994
  Bottom 0: 80.41,51.87 80.1,51.87
S$14995
  Bottom 0: 80.1,51.87 79.79,51.78
S$14996
  Bottom 0: 79.79,51.78 79.51,51.6
S$14997
  Bottom 0: 79.51,51.6 79.3,51.36
S$14998
  Bottom 0: 79.3,51.36 79.16,51.06
S$14999
  Bottom 0: 79.16,51.06 79.12,50.74
S$15000
  Bottom 0: 79.12,50.74 79.16,50.42
S$15001
  Bottom 0: 79.16,50.42 79.3,50.11
S$15002
  Bottom 0: 79.3,50.11 79.51,49.87
S$15003
  Bottom 0: 79.51,49.87 79.79,49.7
S$15004
  Bottom 0: 79.79,49.7 80.1,49.6
S$15005
  Bottom 0: 80.1,49.6 80.42,49.6
S$15006
  Bottom 0: 80.42,49.6 80.73,49.7
S$15007
  Bottom 0: 80.73,49.7 81.01,49.87
S$15008
  Bottom 0: 81.01,49.87 81.22,50.11
S$15009
  Bottom 0: 81.22,50.11 81.28,50.26
S$15010
  Bottom 0: 81.28,50.26 81.28,46.3
S$15011
  Bottom 0: 81.28,46.3 81.2,46.21
S$15012
  Bottom 0: 81.2,46.21 81.1,46.53
S$15013
  Bottom 0: 81.1,46.53 80.89,46.93
S$15014
  Bottom 0: 80.89,46.93 80.61,47.27
S$15015
  Bottom 0: 80.61,47.27 80.26,47.56
S$15016
  Bottom 0: 80.26,47.56 79.86,47.77
S$15017
  Bottom 0: 79.86,47.77 79.44,47.89
S$15018
  Bottom 0: 79.44,47.89 78.99,47.94
S$15019
  Bottom 0: 78.99,47.94 78.54,47.89
S$15020
  Bottom 0: 78.54,47.89 78.11,47.77
S$15021
  Bottom 0: 78.11,47.77 77.72,47.56
S$15022
  Bottom 0: 77.72,47.56 77.38,47.27
S$15023
  Bottom 0: 77.38,47.27 77.09,46.93
S$15024
  Bottom 0: 77.09,46.93 76.88,46.53
S$15025
  Bottom 0: 76.88,46.53 76.75,46.1
S$15026
  Bottom 0: 76.75,46.1 76.7,45.66
S$15027
  Bottom 0: 76.7,45.66 76.75,45.21
S$15028
  Bottom 0: 76.75,45.21 76.84,44.92
S$15029
  Bottom 0: 76.83,49.59 78.61,49.59
S$15030
  Bottom 0: 78.61,49.59 78.68,49.6
S$15031
  Bottom 0: 78.68,49.6 78.76,49.64
S$15032
  Bottom 0: 78.76,49.64 78.81,49.7
S$15033
  Bottom 0: 78.81,49.7 78.85,49.77
S$15034
  Bottom 0: 78.85,49.77 78.86,49.85
S$15035
  Bottom 0: 78.86,49.85 78.86,51.63
S$15036
  Bottom 0: 78.86,51.63 78.85,51.7
S$15037
  Bottom 0: 78.85,51.7 78.81,51.77
S$15038
  Bottom 0: 78.81,51.77 78.76,51.83
S$15039
  Bottom 0: 78.76,51.83 78.68,51.87
S$15040
  Bottom 0: 78.68,51.87 78.61,51.88
S$15041
  Bottom 0: 78.61,51.88 78.16,51.88
S$15042
  Bottom 0: 78.16,51.88 78.16,52.01
S$15043
  Bottom 0: 78.16,52.01 78.1,52.23
S$15044
  Bottom 0: 78.1,52.23 77.94,52.39
S$15045
  Bottom 0: 77.94,52.39 77.72,52.45
S$15046
  Bottom 0: 77.72,52.45 77.37,52.45
S$15047
  Bottom 0: 77.37,52.45 76.28,53.54
S$15048
  Bottom 0: 76.28,53.54 76.34,53.67
S$15049
  Bottom 0: 76.34,53.67 76.39,53.99
S$15050
  Bottom 0: 76.39,53.99 76.34,54.31
S$15051
  Bottom 0: 76.34,54.31 76.21,54.61
S$15052
  Bottom 0: 76.21,54.61 76,54.87
S$15053
  Bottom 0: 76,54.87 75.74,55.05
S$15054
  Bottom 0: 75.74,55.05 75.44,55.16
S$15055
  Bottom 0: 75.44,55.16 75.11,55.18
S$15056
  Bottom 0: 75.11,55.18 74.79,55.12
S$15057
  Bottom 0: 74.79,55.12 74.5,54.97
S$15058
  Bottom 0: 74.5,54.97 74.27,54.74
S$15059
  Bottom 0: 74.27,54.74 74.09,54.47
S$15060
  Bottom 0: 74.09,54.47 74.01,54.16
S$15061
  Bottom 0: 74.01,54.16 74.01,53.83
S$15062
  Bottom 0: 74.01,53.83 74.09,53.52
S$15063
  Bottom 0: 74.09,53.52 74.27,53.24
S$15064
  Bottom 0: 74.27,53.24 74.5,53.02
S$15065
  Bottom 0: 74.5,53.02 74.79,52.87
S$15066
  Bottom 0: 74.79,52.87 75.11,52.8
S$15067
  Bottom 0: 75.11,52.8 75.44,52.82
S$15068
  Bottom 0: 75.44,52.82 75.65,52.9
S$15069
  Bottom 0: 75.65,52.9 76.71,51.84
S$15070
  Bottom 0: 76.71,51.84 76.68,51.83
S$15071
  Bottom 0: 76.68,51.83 76.63,51.77
S$15072
  Bottom 0: 76.63,51.77 76.59,51.7
S$15073
  Bottom 0: 76.59,51.7 76.58,51.63
S$15074
  Bottom 0: 76.58,51.63 76.58,49.85
S$15075
  Bottom 0: 76.58,49.85 76.59,49.77
S$15076
  Bottom 0: 76.59,49.77 76.63,49.7
S$15077
  Bottom 0: 76.63,49.7 76.68,49.64
S$15078
  Bottom 0: 76.68,49.64 76.76,49.6
S$15079
  Bottom 0: 76.76,49.6 76.83,49.59
S$15080
  Bottom 0: 82.24,46.26 82.17,46.31
S$15081
  Bottom 0: 82.17,46.31 82.17,51.18
S$15082
  Bottom 0: 82.17,51.18 82.17,51.25
S$15083
  Bottom 0: 82.17,51.25 82.15,51.32
S$15084
  Bottom 0: 82.15,51.32 82.13,51.38
S$15085
  Bottom 0: 82.13,51.38 82.08,51.44
S$15086
  Bottom 0: 82.08,51.44 82.05,51.49
S$15087
  Bottom 0: 82.05,51.49 75.02,58.51
S$15088
  Bottom 0: 75.02,58.51 77.42,60.92
S$15089
  Bottom 0: 77.42,60.92 77.44,60.9
S$15090
  Bottom 0: 77.44,60.9 77.78,60.8
S$15091
  Bottom 0: 77.78,60.8 78.13,60.77
S$15092
  Bottom 0: 78.13,60.77 78.47,60.84
S$15093
  Bottom 0: 78.47,60.84 78.79,60.99
S$15094
  Bottom 0: 78.79,60.99 79.06,61.21
S$15095
  Bottom 0: 79.06,61.21 79.27,61.5
S$15096
  Bottom 0: 79.27,61.5 79.39,61.82
S$15097
  Bottom 0: 79.39,61.82 79.44,62.17
S$15098
  Bottom 0: 79.44,62.17 79.42,62.29
S$15099
  Bottom 0: 79.42,62.29 83.72,58
S$15100
  Bottom 0: 83.72,58 83.72,54.75
S$15101
  Bottom 0: 83.72,54.75 83.62,54.87
S$15102
  Bottom 0: 83.62,54.87 83.36,55.05
S$15103
  Bottom 0: 83.36,55.05 83.06,55.16
S$15104
  Bottom 0: 83.06,55.16 82.73,55.18
S$15105
  Bottom 0: 82.73,55.18 82.41,55.12
S$15106
  Bottom 0: 82.41,55.12 82.12,54.97
S$15107
  Bottom 0: 82.12,54.97 81.89,54.74
S$15108
  Bottom 0: 81.89,54.74 81.71,54.47
S$15109
  Bottom 0: 81.71,54.47 81.63,54.16
S$15110
  Bottom 0: 81.63,54.16 81.63,53.83
S$15111
  Bottom 0: 81.63,53.83 81.71,53.52
S$15112
  Bottom 0: 81.71,53.52 81.89,53.24
S$15113
  Bottom 0: 81.89,53.24 82.12,53.02
S$15114
  Bottom 0: 82.12,53.02 82.24,52.96
S$15115
  Bottom 0: 82.24,52.96 82.24,46.26
S$15116
  Bottom 0: 49.49,49.32 46.9,51.91
S$15117
  Bottom 0: 46.9,51.91 46.9,53.95
S$15118
  Bottom 0: 46.9,53.95 46.97,53.99
S$15119
  Bottom 0: 46.97,53.99 47.1,54.21
S$15120
  Bottom 0: 47.1,54.21 47.15,54.46
S$15121
  Bottom 0: 47.15,54.46 47.1,54.71
S$15122
  Bottom 0: 47.1,54.71 46.98,54.91
S$15123
  Bottom 0: 46.98,54.91 55.4,54.91
S$15124
  Bottom 0: 55.4,54.91 55.22,54.74
S$15125
  Bottom 0: 55.22,54.74 55.04,54.47
S$15126
  Bottom 0: 55.04,54.47 54.96,54.15
S$15127
  Bottom 0: 54.96,54.15 54.96,53.83
S$15128
  Bottom 0: 54.96,53.83 55.04,53.51
S$15129
  Bottom 0: 55.04,53.51 55.22,53.23
S$15130
  Bottom 0: 55.22,53.23 55.45,53.01
S$15131
  Bottom 0: 55.45,53.01 55.74,52.87
S$15132
  Bottom 0: 55.74,52.87 56.06,52.8
S$15133
  Bottom 0: 56.06,52.8 56.38,52.82
S$15134
  Bottom 0: 56.38,52.82 56.6,52.9
S$15135
  Bottom 0: 56.6,52.9 57.66,51.84
S$15136
  Bottom 0: 57.66,51.84 57.64,51.83
S$15137
  Bottom 0: 57.64,51.83 57.58,51.77
S$15138
  Bottom 0: 57.58,51.77 57.54,51.7
S$15139
  Bottom 0: 57.54,51.7 57.53,51.63
S$15140
  Bottom 0: 57.53,51.63 57.53,49.83
S$15141
  Bottom 0: 57.53,49.83 51.41,49.83
S$15142
  Bottom 0: 51.41,49.83 51.39,50
S$15143
  Bottom 0: 51.39,50 51.26,50.27
S$15144
  Bottom 0: 51.26,50.27 51.06,50.49
S$15145
  Bottom 0: 51.06,50.49 50.79,50.65
S$15146
  Bottom 0: 50.79,50.65 50.49,50.71
S$15147
  Bottom 0: 50.49,50.71 50.19,50.69
S$15148
  Bottom 0: 50.19,50.69 49.91,50.58
S$15149
  Bottom 0: 49.91,50.58 49.67,50.39
S$15150
  Bottom 0: 49.67,50.39 49.51,50.14
S$15151
  Bottom 0: 49.51,50.14 49.41,49.85
S$15152
  Bottom 0: 49.41,49.85 49.41,49.55
S$15153
  Bottom 0: 49.41,49.55 49.49,49.32
S$15154
  Bottom 0: 146.69,49.72 146.65,50
S$15155
  Bottom 0: 146.65,50 146.51,50.27
S$15156
  Bottom 0: 146.51,50.27 146.31,50.49
S$15157
  Bottom 0: 146.31,50.49 146.05,50.65
S$15158
  Bottom 0: 146.05,50.65 145.75,50.71
S$15159
  Bottom 0: 145.75,50.71 145.45,50.69
S$15160
  Bottom 0: 145.45,50.69 145.17,50.58
S$15161
  Bottom 0: 145.17,50.58 144.93,50.39
S$15162
  Bottom 0: 144.93,50.39 144.76,50.14
S$15163
  Bottom 0: 144.76,50.14 144.68,49.88
S$15164
  Bottom 0: 144.68,49.88 138.17,49.88
S$15165
  Bottom 0: 138.17,49.88 138.37,50.11
S$15166
  Bottom 0: 138.37,50.11 138.51,50.42
S$15167
  Bottom 0: 138.51,50.42 138.55,50.74
S$15168
  Bottom 0: 138.55,50.74 138.51,51.06
S$15169
  Bottom 0: 138.51,51.06 138.37,51.36
S$15170
  Bottom 0: 138.37,51.36 138.16,51.6
S$15171
  Bottom 0: 138.16,51.6 137.98,51.72
S$15172
  Bottom 0: 137.98,51.72 137.98,55.26
S$15173
  Bottom 0: 137.98,55.26 147.08,64.37
S$15174
  Bottom 0: 147.08,64.37 148.35,65.63
S$15175
  Bottom 0: 148.35,65.63 148.32,65.58
S$15176
  Bottom 0: 148.32,65.58 148.19,65.15
S$15177
  Bottom 0: 148.19,65.15 148.15,64.71
S$15178
  Bottom 0: 148.15,64.71 148.19,64.26
S$15179
  Bottom 0: 148.19,64.26 148.32,63.83
S$15180
  Bottom 0: 148.32,63.83 148.53,63.44
S$15181
  Bottom 0: 148.53,63.44 148.82,63.09
S$15182
  Bottom 0: 148.82,63.09 149.16,62.81
S$15183
  Bottom 0: 149.16,62.81 149.56,62.59
S$15184
  Bottom 0: 149.56,62.59 149.98,62.47
S$15185
  Bottom 0: 149.98,62.47 150.43,62.42
S$15186
  Bottom 0: 150.43,62.42 150.88,62.47
S$15187
  Bottom 0: 150.88,62.47 151.18,62.56
S$15188
  Bottom 0: 151.18,62.56 150.17,61.54
S$15189
  Bottom 0: 150.17,61.54 150.12,61.49
S$15190
  Bottom 0: 150.12,61.49 150.09,61.44
S$15191
  Bottom 0: 150.09,61.44 150.06,61.37
S$15192
  Bottom 0: 150.06,61.37 150.04,61.3
S$15193
  Bottom 0: 150.04,61.3 150.03,61.23
S$15194
  Bottom 0: 150.03,61.23 150.03,58.99
S$15195
  Bottom 0: 150.03,58.99 147.66,56.61
S$15196
  Bottom 0: 147.66,56.61 147.62,56.56
S$15197
  Bottom 0: 147.62,56.56 147.58,56.5
S$15198
  Bottom 0: 147.58,56.5 147.55,56.44
S$15199
  Bottom 0: 147.55,56.44 147.54,56.37
S$15200
  Bottom 0: 147.54,56.37 147.54,56.3
S$15201
  Bottom 0: 147.54,56.3 147.54,50.57
S$15202
  Bottom 0: 147.54,50.57 146.69,49.72
S$15203
  Bottom 0: 139.88,52.8 140.21,52.82
S$15204
  Bottom 0: 140.21,52.82 140.51,52.93
S$15205
  Bottom 0: 140.51,52.93 140.78,53.12
S$15206
  Bottom 0: 140.78,53.12 140.99,53.37
S$15207
  Bottom 0: 140.99,53.37 141.12,53.67
S$15208
  Bottom 0: 141.12,53.67 141.16,53.99
S$15209
  Bottom 0: 141.16,53.99 141.12,54.31
S$15210
  Bottom 0: 141.12,54.31 140.99,54.61
S$15211
  Bottom 0: 140.99,54.61 140.78,54.87
S$15212
  Bottom 0: 140.78,54.87 140.51,55.05
S$15213
  Bottom 0: 140.51,55.05 140.21,55.16
S$15214
  Bottom 0: 140.21,55.16 139.88,55.18
S$15215
  Bottom 0: 139.88,55.18 139.56,55.12
S$15216
  Bottom 0: 139.56,55.12 139.28,54.97
S$15217
  Bottom 0: 139.28,54.97 139.04,54.74
S$15218
  Bottom 0: 139.04,54.74 138.87,54.47
S$15219
  Bottom 0: 138.87,54.47 138.78,54.16
S$15220
  Bottom 0: 138.78,54.16 138.78,53.83
S$15221
  Bottom 0: 138.78,53.83 138.87,53.52
S$15222
  Bottom 0: 138.87,53.52 139.04,53.24
S$15223
  Bottom 0: 139.04,53.24 139.28,53.02
S$15224
  Bottom 0: 139.28,53.02 139.56,52.87
S$15225
  Bottom 0: 139.56,52.87 139.88,52.8
S$15226
  Bottom 0: 147.98,58.23 148.32,58.3
S$15227
  Bottom 0: 148.32,58.3 148.64,58.45
S$15228
  Bottom 0: 148.64,58.45 148.91,58.67
S$15229
  Bottom 0: 148.91,58.67 149.12,58.96
S$15230
  Bottom 0: 149.12,58.96 149.24,59.28
S$15231
  Bottom 0: 149.24,59.28 149.29,59.63
S$15232
  Bottom 0: 149.29,59.63 149.24,59.97
S$15233
  Bottom 0: 149.24,59.97 149.12,60.3
S$15234
  Bottom 0: 149.12,60.3 148.91,60.58
S$15235
  Bottom 0: 148.91,60.58 148.64,60.8
S$15236
  Bottom 0: 148.64,60.8 148.32,60.96
S$15237
  Bottom 0: 148.32,60.96 147.98,61.02
S$15238
  Bottom 0: 147.98,61.02 147.63,61
S$15239
  Bottom 0: 147.63,61 147.3,60.89
S$15240
  Bottom 0: 147.3,60.89 147,60.7
S$15241
  Bottom 0: 147,60.7 146.76,60.45
S$15242
  Bottom 0: 146.76,60.45 146.59,60.14
S$15243
  Bottom 0: 146.59,60.14 146.5,59.8
S$15244
  Bottom 0: 146.5,59.8 146.5,59.45
S$15245
  Bottom 0: 146.5,59.45 146.59,59.11
S$15246
  Bottom 0: 146.59,59.11 146.76,58.8
S$15247
  Bottom 0: 146.76,58.8 147,58.55
S$15248
  Bottom 0: 147,58.55 147.3,58.36
S$15249
  Bottom 0: 147.3,58.36 147.63,58.26
S$15250
  Bottom 0: 147.63,58.26 147.98,58.23
S$15251
  Bottom 0: 59.82,49.83 59.82,51.63
S$15252
  Bottom 0: 59.82,51.63 59.81,51.7
S$15253
  Bottom 0: 59.81,51.7 59.77,51.77
S$15254
  Bottom 0: 59.77,51.77 59.71,51.83
S$15255
  Bottom 0: 59.71,51.83 59.64,51.87
S$15256
  Bottom 0: 59.64,51.87 59.57,51.88
S$15257
  Bottom 0: 59.57,51.88 59.12,51.88
S$15258
  Bottom 0: 59.12,51.88 59.12,52.01
S$15259
  Bottom 0: 59.12,52.01 59.06,52.23
S$15260
  Bottom 0: 59.06,52.23 58.9,52.39
S$15261
  Bottom 0: 58.9,52.39 58.68,52.45
S$15262
  Bottom 0: 58.68,52.45 58.31,52.45
S$15263
  Bottom 0: 58.31,52.45 57.23,53.53
S$15264
  Bottom 0: 57.23,53.53 57.29,53.67
S$15265
  Bottom 0: 57.29,53.67 57.34,53.98
S$15266
  Bottom 0: 57.34,53.98 57.29,54.3
S$15267
  Bottom 0: 57.29,54.3 57.16,54.61
S$15268
  Bottom 0: 57.16,54.61 56.95,54.86
S$15269
  Bottom 0: 56.95,54.86 56.89,54.91
S$15270
  Bottom 0: 56.89,54.91 62.04,54.91
S$15271
  Bottom 0: 62.04,54.91 62.62,54.32
S$15272
  Bottom 0: 62.62,54.32 62.58,54.15
S$15273
  Bottom 0: 62.58,54.15 62.58,53.83
S$15274
  Bottom 0: 62.58,53.83 62.66,53.51
S$15275
  Bottom 0: 62.66,53.51 62.84,53.23
S$15276
  Bottom 0: 62.84,53.23 63.07,53.01
S$15277
  Bottom 0: 63.07,53.01 63.36,52.87
S$15278
  Bottom 0: 63.36,52.87 63.68,52.8
S$15279
  Bottom 0: 63.68,52.8 64,52.82
S$15280
  Bottom 0: 64,52.82 64.31,52.93
S$15281
  Bottom 0: 64.31,52.93 64.57,53.11
S$15282
  Bottom 0: 64.57,53.11 64.78,53.37
S$15283
  Bottom 0: 64.78,53.37 64.8,53.42
S$15284
  Bottom 0: 64.8,53.42 66.73,53.42
S$15285
  Bottom 0: 66.73,53.42 69.44,50.71
S$15286
  Bottom 0: 69.44,50.71 69.24,50.69
S$15287
  Bottom 0: 69.24,50.69 68.96,50.58
S$15288
  Bottom 0: 68.96,50.58 68.72,50.39
S$15289
  Bottom 0: 68.72,50.39 68.56,50.14
S$15290
  Bottom 0: 68.56,50.14 68.46,49.85
S$15291
  Bottom 0: 68.46,49.85 68.46,49.83
S$15292
  Bottom 0: 68.46,49.83 61.9,49.83
S$15293
  Bottom 0: 61.9,49.83 61.96,49.87
S$15294
  Bottom 0: 61.96,49.87 62.17,50.11
S$15295
  Bottom 0: 62.17,50.11 62.31,50.42
S$15296
  Bottom 0: 62.31,50.42 62.36,50.74
S$15297
  Bottom 0: 62.36,50.74 62.31,51.06
S$15298
  Bottom 0: 62.31,51.06 62.17,51.36
S$15299
  Bottom 0: 62.17,51.36 61.96,51.6
S$15300
  Bottom 0: 61.96,51.6 61.69,51.78
S$15301
  Bottom 0: 61.69,51.78 61.38,51.87
S$15302
  Bottom 0: 61.38,51.87 61.05,51.87
S$15303
  Bottom 0: 61.05,51.87 60.74,51.78
S$15304
  Bottom 0: 60.74,51.78 60.47,51.6
S$15305
  Bottom 0: 60.47,51.6 60.26,51.36
S$15306
  Bottom 0: 60.26,51.36 60.12,51.06
S$15307
  Bottom 0: 60.12,51.06 60.07,50.74
S$15308
  Bottom 0: 60.07,50.74 60.12,50.42
S$15309
  Bottom 0: 60.12,50.42 60.26,50.11
S$15310
  Bottom 0: 60.26,50.11 60.47,49.87
S$15311
  Bottom 0: 60.47,49.87 60.53,49.83
S$15312
  Bottom 0: 60.53,49.83 59.82,49.83
S$15313
  Bottom 0: 155.06,50.14 155.06,51.63
S$15314
  Bottom 0: 155.06,51.63 155.05,51.7
S$15315
  Bottom 0: 155.05,51.7 155.01,51.77
S$15316
  Bottom 0: 155.01,51.77 154.96,51.83
S$15317
  Bottom 0: 154.96,51.83 154.89,51.87
S$15318
  Bottom 0: 154.89,51.87 154.81,51.88
S$15319
  Bottom 0: 154.81,51.88 154.36,51.88
S$15320
  Bottom 0: 154.36,51.88 154.36,52.01
S$15321
  Bottom 0: 154.36,52.01 154.3,52.23
S$15322
  Bottom 0: 154.3,52.23 154.14,52.39
S$15323
  Bottom 0: 154.14,52.39 153.92,52.45
S$15324
  Bottom 0: 153.92,52.45 153.58,52.45
S$15325
  Bottom 0: 153.58,52.45 152.49,53.54
S$15326
  Bottom 0: 152.49,53.54 152.55,53.67
S$15327
  Bottom 0: 152.55,53.67 152.6,53.99
S$15328
  Bottom 0: 152.6,53.99 152.55,54.31
S$15329
  Bottom 0: 152.55,54.31 152.42,54.61
S$15330
  Bottom 0: 152.42,54.61 152.22,54.87
S$15331
  Bottom 0: 152.22,54.87 151.95,55.05
S$15332
  Bottom 0: 151.95,55.05 151.65,55.16
S$15333
  Bottom 0: 151.65,55.16 151.32,55.18
S$15334
  Bottom 0: 151.32,55.18 151.24,55.17
S$15335
  Bottom 0: 151.24,55.17 157.58,61.51
S$15336
  Bottom 0: 157.58,61.51 157.97,61.51
S$15337
  Bottom 0: 157.97,61.51 158.05,61.51
S$15338
  Bottom 0: 158.05,61.51 158.11,61.53
S$15339
  Bottom 0: 158.11,61.53 158.17,61.55
S$15340
  Bottom 0: 158.17,61.55 158.23,61.59
S$15341
  Bottom 0: 158.23,61.59 158.29,61.63
S$15342
  Bottom 0: 158.29,61.63 158.49,61.83
S$15343
  Bottom 0: 158.49,61.83 158.52,61.83
S$15344
  Bottom 0: 158.52,61.83 158.59,61.82
S$15345
  Bottom 0: 158.59,61.82 159.22,61.82
S$15346
  Bottom 0: 159.22,61.82 159.06,61.57
S$15347
  Bottom 0: 159.06,61.57 158.97,61.28
S$15348
  Bottom 0: 158.97,61.28 158.97,60.98
S$15349
  Bottom 0: 158.97,60.98 159.06,60.69
S$15350
  Bottom 0: 159.06,60.69 159.22,60.44
S$15351
  Bottom 0: 159.22,60.44 159.46,60.25
S$15352
  Bottom 0: 159.46,60.25 159.74,60.14
S$15353
  Bottom 0: 159.74,60.14 160.05,60.12
S$15354
  Bottom 0: 160.05,60.12 160.34,60.19
S$15355
  Bottom 0: 160.34,60.19 160.6,60.34
S$15356
  Bottom 0: 160.6,60.34 160.81,60.56
S$15357
  Bottom 0: 160.81,60.56 160.94,60.83
S$15358
  Bottom 0: 160.94,60.83 160.99,61.13
S$15359
  Bottom 0: 160.99,61.13 160.94,61.43
S$15360
  Bottom 0: 160.94,61.43 160.81,61.7
S$15361
  Bottom 0: 160.81,61.7 160.7,61.82
S$15362
  Bottom 0: 160.7,61.82 170.77,61.82
S$15363
  Bottom 0: 170.77,61.82 170.85,61.83
S$15364
  Bottom 0: 170.85,61.83 170.91,61.84
S$15365
  Bottom 0: 170.91,61.84 170.97,61.86
S$15366
  Bottom 0: 170.97,61.86 171.03,61.91
S$15367
  Bottom 0: 171.03,61.91 171.09,61.95
S$15368
  Bottom 0: 171.09,61.95 172.41,63.27
S$15369
  Bottom 0: 172.41,63.27 172.44,63.27
S$15370
  Bottom 0: 172.44,63.27 172.4,63.24
S$15371
  Bottom 0: 172.4,63.24 172.16,62.99
S$15372
  Bottom 0: 172.16,62.99 171.99,62.68
S$15373
  Bottom 0: 171.99,62.68 171.91,62.34
S$15374
  Bottom 0: 171.91,62.34 171.91,61.99
S$15375
  Bottom 0: 171.91,61.99 171.99,61.65
S$15376
  Bottom 0: 171.99,61.65 172.04,61.55
S$15377
  Bottom 0: 172.04,61.55 168.92,58.43
S$15378
  Bottom 0: 168.92,58.43 167.65,58.43
S$15379
  Bottom 0: 167.65,58.43 167.69,58.45
S$15380
  Bottom 0: 167.69,58.45 167.96,58.67
S$15381
  Bottom 0: 167.96,58.67 168.17,58.96
S$15382
  Bottom 0: 168.17,58.96 168.29,59.28
S$15383
  Bottom 0: 168.29,59.28 168.34,59.63
S$15384
  Bottom 0: 168.34,59.63 168.29,59.97
S$15385
  Bottom 0: 168.29,59.97 168.17,60.3
S$15386
  Bottom 0: 168.17,60.3 167.96,60.58
S$15387
  Bottom 0: 167.96,60.58 167.69,60.8
S$15388
  Bottom 0: 167.69,60.8 167.37,60.96
S$15389
  Bottom 0: 167.37,60.96 167.03,61.02
S$15390
  Bottom 0: 167.03,61.02 166.68,61
S$15391
  Bottom 0: 166.68,61 166.35,60.89
S$15392
  Bottom 0: 166.35,60.89 166.05,60.7
S$15393
  Bottom 0: 166.05,60.7 165.81,60.45
S$15394
  Bottom 0: 165.81,60.45 165.64,60.14
S$15395
  Bottom 0: 165.64,60.14 165.56,59.8
S$15396
  Bottom 0: 165.56,59.8 165.56,59.45
S$15397
  Bottom 0: 165.56,59.45 165.64,59.11
S$15398
  Bottom 0: 165.64,59.11 165.81,58.8
S$15399
  Bottom 0: 165.81,58.8 166.05,58.55
S$15400
  Bottom 0: 166.05,58.55 166.25,58.43
S$15401
  Bottom 0: 166.25,58.43 156.25,58.43
S$15402
  Bottom 0: 156.25,58.43 156.18,58.42
S$15403
  Bottom 0: 156.18,58.42 156.11,58.41
S$15404
  Bottom 0: 156.11,58.41 156.05,58.38
S$15405
  Bottom 0: 156.05,58.38 155.99,58.34
S$15406
  Bottom 0: 155.99,58.34 155.94,58.3
S$15407
  Bottom 0: 155.94,58.3 154.17,56.53
S$15408
  Bottom 0: 154.17,56.53 154.12,56.48
S$15409
  Bottom 0: 154.12,56.48 154.09,56.43
S$15410
  Bottom 0: 154.09,56.43 154.06,56.36
S$15411
  Bottom 0: 154.06,56.36 154.04,56.29
S$15412
  Bottom 0: 154.04,56.29 154.04,56.22
S$15413
  Bottom 0: 154.04,56.22 154.04,54.93
S$15414
  Bottom 0: 154.04,54.93 154.04,54.86
S$15415
  Bottom 0: 154.04,54.86 154.06,54.79
S$15416
  Bottom 0: 154.06,54.79 154.08,54.73
S$15417
  Bottom 0: 154.08,54.73 154.12,54.67
S$15418
  Bottom 0: 154.12,54.67 154.16,54.61
S$15419
  Bottom 0: 154.16,54.61 157.12,51.66
S$15420
  Bottom 0: 157.12,51.66 156.93,51.78
S$15421
  Bottom 0: 156.93,51.78 156.62,51.87
S$15422
  Bottom 0: 156.62,51.87 156.3,51.87
S$15423
  Bottom 0: 156.3,51.87 155.99,51.78
S$15424
  Bottom 0: 155.99,51.78 155.71,51.6
S$15425
  Bottom 0: 155.71,51.6 155.5,51.36
S$15426
  Bottom 0: 155.5,51.36 155.36,51.06
S$15427
  Bottom 0: 155.36,51.06 155.32,50.74
S$15428
  Bottom 0: 155.32,50.74 155.36,50.43
S$15429
  Bottom 0: 155.36,50.43 155.06,50.14
S$15430
  Bottom 0: 241.11,52.41 241.1,52.42
S$15431
  Bottom 0: 241.1,52.42 241.03,52.43
S$15432
  Bottom 0: 241.03,52.43 240.96,52.44
S$15433
  Bottom 0: 240.96,52.44 223.87,52.44
S$15434
  Bottom 0: 223.87,52.44 208.26,68.05
S$15435
  Bottom 0: 208.26,68.05 211.34,68.05
S$15436
  Bottom 0: 211.34,68.05 217.27,62.13
S$15437
  Bottom 0: 217.27,62.13 217.19,62.14
S$15438
  Bottom 0: 217.19,62.14 216.89,62.12
S$15439
  Bottom 0: 216.89,62.12 216.61,62.01
S$15440
  Bottom 0: 216.61,62.01 216.37,61.82
S$15441
  Bottom 0: 216.37,61.82 216.21,61.57
S$15442
  Bottom 0: 216.21,61.57 216.11,61.28
S$15443
  Bottom 0: 216.11,61.28 216.11,60.98
S$15444
  Bottom 0: 216.11,60.98 216.21,60.69
S$15445
  Bottom 0: 216.21,60.69 216.37,60.44
S$15446
  Bottom 0: 216.37,60.44 216.61,60.25
S$15447
  Bottom 0: 216.61,60.25 216.89,60.14
S$15448
  Bottom 0: 216.89,60.14 217.19,60.12
S$15449
  Bottom 0: 217.19,60.12 217.49,60.19
S$15450
  Bottom 0: 217.49,60.19 217.76,60.34
S$15451
  Bottom 0: 217.76,60.34 217.96,60.56
S$15452
  Bottom 0: 217.96,60.56 218.02,60.69
S$15453
  Bottom 0: 218.02,60.69 222.4,60.69
S$15454
  Bottom 0: 222.4,60.69 222.84,60.24
S$15455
